FUNCTION FC 8 : VOID
TITLE =COMANDI PROFIBUS AZIONAMENTO 8 NASTRI
VERSION : 0.1

BEGIN
NETWORK
TITLE =TRASFERISCO I SEGNALI DI COMANDO
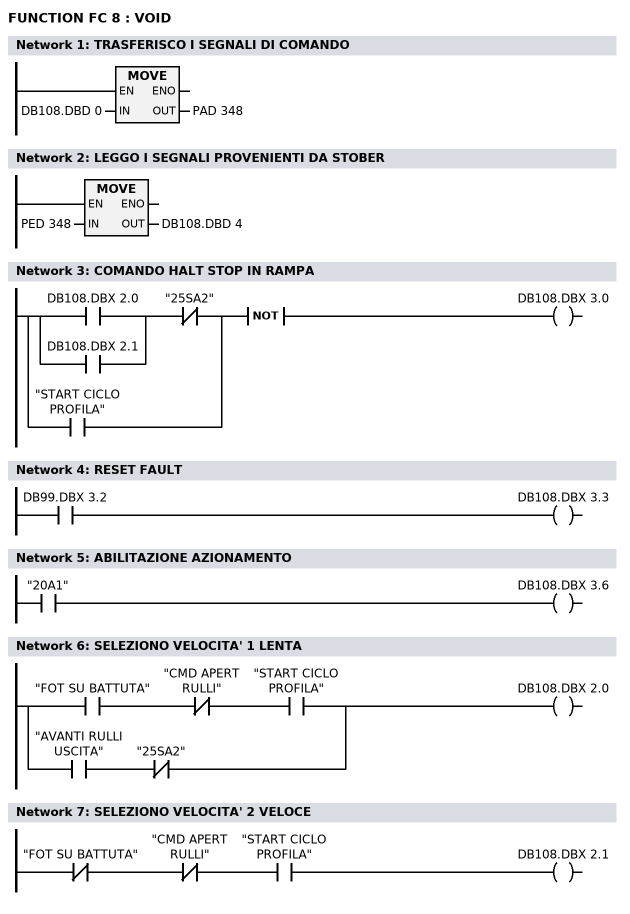
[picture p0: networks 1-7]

      L     DB108.DBD    0;
      T     PAD  348;
      NOP   0;
NETWORK
TITLE =LEGGO I SEGNALI PROVENIENTI DA STOBER

      L     PED  348;
      T     DB108.DBD    4;
      NOP   0;
NETWORK
TITLE =COMANDO HALT STOP IN RAMPA

      U     DB108.DBX    2.0;
      O     DB108.DBX    2.1;
      UN    "25SA2";
      O     "START CICLO PROFILA";
      NOT   ;
      =     DB108.DBX    3.0;
NETWORK
TITLE =RESET FAULT

      U     DB99.DBX    3.2;
      =     DB108.DBX    3.3;
NETWORK
TITLE =ABILITAZIONE AZIONAMENTO

      U     "20A1";
      =     DB108.DBX    3.6;
NETWORK
TITLE =SELEZIONO VELOCITA' 1 LENTA

      U     "FOT SU BATTUTA";
      UN    "CMD APERT RULLI";
      U     "START CICLO PROFILA";
      O     ;
      U     "AVANTI RULLI USCITA";
      UN    "25SA2";
      =     DB108.DBX    2.0;
NETWORK
TITLE =SELEZIONO VELOCITA' 2 VELOCE

      UN    "FOT SU BATTUTA";
      UN    "CMD APERT RULLI";
      U     "START CICLO PROFILA";
      =     DB108.DBX    2.1;

END_FUNCTION

